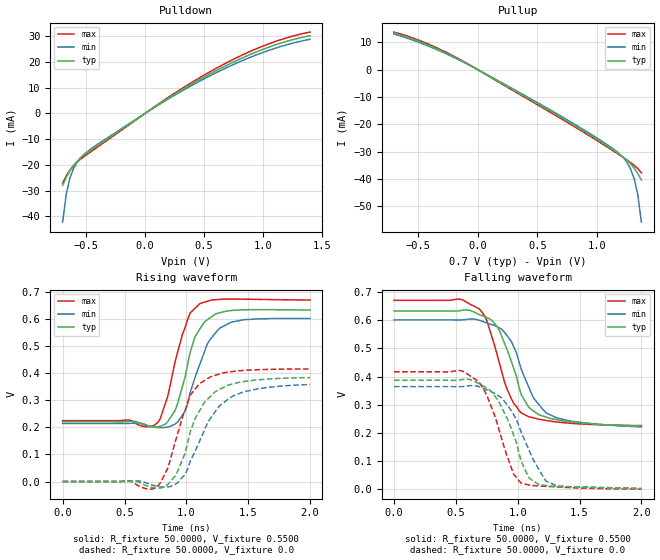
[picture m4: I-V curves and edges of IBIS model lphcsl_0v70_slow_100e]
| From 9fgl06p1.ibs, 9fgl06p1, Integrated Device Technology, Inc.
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[Model]   lphcsl_0v70_slow_100e
Model_type Output
Polarity   Non-Inverting
Enable   Active-High
Vmeas =  0.4000V
Cref =   2.0000pF
Rref =   0.0
Vref =   0.4000V
C_comp   1.1000pF   1.0000pF   1.2000pF
[Temperature Range]   25.0000   85.0000   -40.0000
[Voltage Range]   0.7000V   0.6700V   0.7400V
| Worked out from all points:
|   slope of the pulldown table from 0 to 0.105 V, typ, clamps not added: 32.9 ohm
|   slope of the pullup table from 0 to 0.105 V, typ, clamps not added: 40.5 ohm
|   rising waveform, R_fixture 50.0000, V_fixture 0.5500: 20-80 % time 153ps typ, 179ps min, 150ps max; typ from 0.221 V to 0.635 V
|   rising waveform, R_fixture 50.0000, V_fixture 0.0: 20-80 % time 214ps typ, 259ps min, 184ps max; typ from 0 V to 0.385 V
|   falling waveform, R_fixture 50.0000, V_fixture 0.5500: 20-80 % time 206ps typ, 230ps min, 193ps max; typ from 0.633 V to 0.224 V
|   falling waveform, R_fixture 50.0000, V_fixture 0.0: 20-80 % time 202ps typ, 238ps min, 192ps max; typ from 0.387 V to 0.002 V
[Pulldown]
|Voltage   I(typ)   I(min)   I(max)
-700mV    -27.91mA   -42.29mA   -27.13mA
-670mV    -24.93mA   -31.58mA   -24.4mA
-640mV    -22.46mA   -25.38mA   -22.16mA
-610mV    -20.43mA   -21.63mA   -20.41mA
-550mV    -17.42mA   -17.37mA   -17.87mA
-460mV    -14.27mA   -13.81mA   -14.87mA
170mV     5.111mA    4.867mA    5.413mA
620mV     17mA       16.18mA    17.92mA
830mV     21.65mA    20.59mA    22.8mA
1.01V     25.07mA    23.84mA    26.32mA
1.22V     28.24mA    26.89mA    29.6mA
1.4V      30.17mA    28.8mA     31.59mA
[Pullup]
|Voltage   I(typ)   I(min)   I(max)
-700mV    13.37mA    12.97mA    13.69mA
-400mV    8.685mA    8.356mA    9.067mA
-40mV     976.3uA    932.1uA    1.037mA
710mV     -17.77mA   -17.34mA   -18.25mA
1.01V     -25.83mA   -25.34mA   -26.25mA
1.16V     -30.15mA   -29.81mA   -30.44mA
1.22V     -32.05mA   -32.24mA   -32.17mA
1.25V     -33.15mA   -33.95mA   -33.06mA
1.28V     -34.44mA   -36.32mA   -33.98mA
1.31V     -36.02mA   -39.87mA   -35mA
1.34V     -37.97mA   -45.72mA   -36.19mA
1.37V     -40.34mA   -55.75mA   -37.7mA
[Ramp]
| variable   typ   min   max
dV/dt_r  0.2309/0.2342n   0.2155/0.2596n   0.2500/0.2037n
dV/dt_f  0.2476/0.2378n   0.2299/0.2670n   0.2694/0.2067n
R_load = 50.0000
[Rising Waveform]
R_fixture= 50.0000
V_fixture= 0.5500
V_fixture_min= 0.5200
V_fixture_max= 0.5800
|time   V(typ)   V(min)   V(max)
0s        221mV      214.9mV    225.3mV
770ps     203.1mV    199.4mV    218.3mV
850ps     221.8mV    201.8mV    315.9mV
910ps     263.8mV    212.8mV    445.4mV
990ps     387.7mV    260.7mV    569.9mV
1.05ns    506.6mV    356.8mV    632.4mV
1.11ns    565.2mV    435.6mV    658.8mV
1.19ns    605.5mV    524.5mV    670mV
1.37ns    633.3mV    590.7mV    675.3mV
2ns       634.9mV    603.3mV    671.9mV
[Rising Waveform]
R_fixture= 50.0000
V_fixture= 0.0
V_fixture_min= 0.0
V_fixture_max= 0.0
|time   V(typ)   V(min)   V(max)
0s        0V         0V         0V
530ps     938.9uV    -3.621uV   2.86mV
730ps     -22.67mV   -13.8mV    -27.79mV
850ps     -10.75mV   -20.27mV   49mV
910ps     20.8mV     -10.8mV    146.5mV
1.03ns    181.5mV    73.41mV    318.8mV
1.11ns    264.6mV    152.6mV    363.3mV
1.25ns    336.9mV    269.8mV    395.6mV
1.37ns    360.5mV    314.9mV    407.1mV
2ns       384.9mV    359.1mV    416.6mV
[Falling Waveform]
R_fixture= 50.0000
V_fixture= 0.5500
V_fixture_min= 0.5200
V_fixture_max= 0.5800
|time   V(typ)   V(min)   V(max)
0s        632.9mV    601.2mV    670.7mV
530ps     633.8mV    601mV      675.2mV
690ps     620.4mV    600mV      640.2mV
750ps     610mV      590.3mV    599.8mV
850ps     566.4mV    573.5mV    451.8mV
950ps     452.4mV    524.2mV    320.5mV
1.03ns    335.6mV    424.4mV    270.8mV
1.13ns    277.8mV    323mV      253.6mV
1.23ns    256.5mV    271.1mV    244.6mV
2ns       224.5mV    221.6mV    226.4mV
[Falling Waveform]
R_fixture= 50.0000
V_fixture= 0.0
V_fixture_min= 0.0
V_fixture_max= 0.0
|time   V(typ)   V(min)   V(max)
0s        387.1mV    364.6mV    417.1mV
530ps     388mV      364.4mV    422mV
690ps     374mV      364mV      379.1mV
750ps     359.8mV    353.2mV    334.4mV
850ps     309.2mV    330.7mV    210.9mV
970ps     189.6mV    263.1mV    52.05mV
1.03ns    98.34mV    201.3mV    22.28mV
1.09ns    41.52mV    141.2mV    15.42mV
1.23ns    13.6mV     28.94mV    10.75mV
2ns       2.235mV    3.662mV    813.5uV
